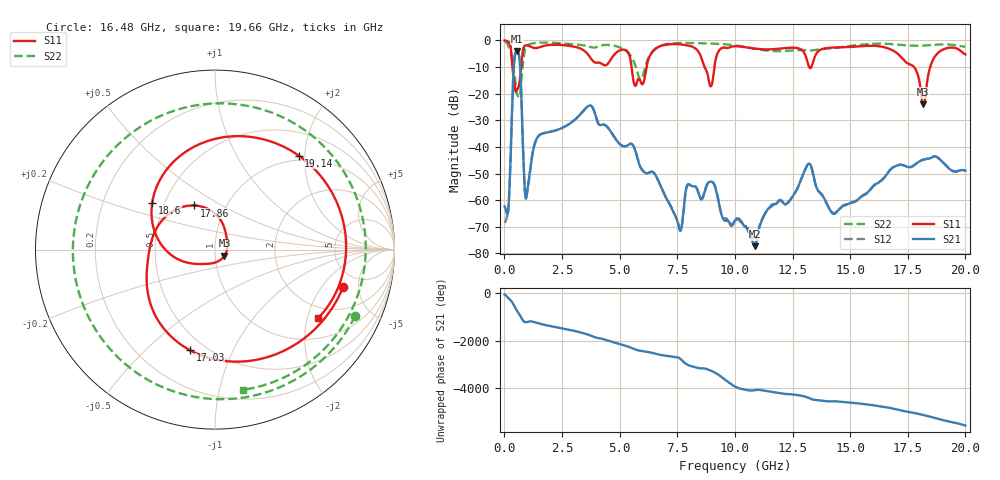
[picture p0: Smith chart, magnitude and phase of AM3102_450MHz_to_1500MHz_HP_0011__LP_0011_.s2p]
!Agilent Technologies,E8364B,MY43040894,A.07.50.67
!Agilent E8364B: A.07.50.67
!Date: Thursday, January 11, 2018 05:30:47
!Correction: S11(Full 2 Port(1,2))
!S21(Full 2 Port(1,2))
!S12(Full 2 Port(1,2))
!S22(Full 2 Port(1,2))
!S2P File: Measurements: S11, S21, S12, S22:
# Hz S  dB  R 50
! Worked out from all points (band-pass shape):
!   1601 points, 10 MHz to 20 GHz, reference 50 ohm
!   highest |S21| = -3.97 dB at 534.7 MHz (marker M1); lowest = -77.3 dB at 10.85 GHz (marker M2)
!   |S21| within 3 dB of the highest: 437.7 MHz to 656 MHz (218.3 MHz wide, 39.9 % of centre)
!   lowest |S11| = -24.0 dB at 18.18 GHz (marker M3), VSWR 1.13, Z = 55.4 - j3.81 ohm
!   |S11| at or under -10 dB: 5.518 GHz to 6.17 GHz (652.1 MHz wide, 11.2 % of centre); 8.684 GHz to 9.111 GHz (426.9 MHz wide, 4.8 % of centre); 17.77 GHz to 18.47 GHz (706.4 MHz wide, 3.9 % of centre)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
!   |S22| runs from -21.4 to -0.4 dB; largest |S21 - S12| = 0.0012
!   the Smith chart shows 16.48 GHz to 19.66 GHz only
!   S11 on the Smith chart (normalised r, x): 16.48 GHz: 3.58, -3.32; 17.03 GHz: 0.41, -0.69; 17.86 GHz: 0.71, +0.38; 18.6 GHz: 0.43, +0.27; 19.14 GHz: 0.91, +1.87; 19.66 GHz: 1.61, -2.34
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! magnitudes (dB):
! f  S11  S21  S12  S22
! 10 MHz  0.0  -62.3  -68.5  -0.4
! 172.4 MHz  -0.6  -63.3  -63.8  -2.1
! 534.7 MHz  -18.6  -4.0  -4.0  -19.7
! 959.5 MHz  -1.9  -58.5  -58.7  -2.2
! 1.459 GHz  -2.8  -36.1  -36.1  -0.9
! 3.346 GHz  -3.3  -27.3  -27.3  -1.8
! 6.682 GHz  -2.5  -52.8  -52.7  -2.4
! 7.619 GHz  -1.5  -71.4  -71.5  -1.0
! 8.956 GHz  -17.3  -53.0  -53.0  -1.2
! 10.01 GHz  -2.2  -67.6  -67.4  -1.9
! 10.85 GHz  -3.1  -77.3  -76.9  -3.1
! 13.34 GHz  -9.6  -48.3  -48.2  -3.8
! 14.3 GHz  -2.7  -65.1  -64.9  -2.9
! 16.48 GHz  -2.6  -51.6  -51.5  -1.3
! 16.68 GHz  -3.1  -49.2  -49.3  -1.3
! 17.03 GHz  -4.8  -47.0  -47.0  -1.6
! 17.86 GHz  -11.3  -46.3  -46.3  -2.0
! 18.18 GHz  -24.0  -44.8  -44.8  -2.0
! 18.6 GHz  -7.2  -43.7  -43.7  -1.7
! 19.14 GHz  -3.1  -46.8  -46.8  -1.5
! 19.66 GHz  -3.2  -49.2  -49.0  -2.0
! 20 GHz  -5.3  -48.9  -49.0  -2.4
